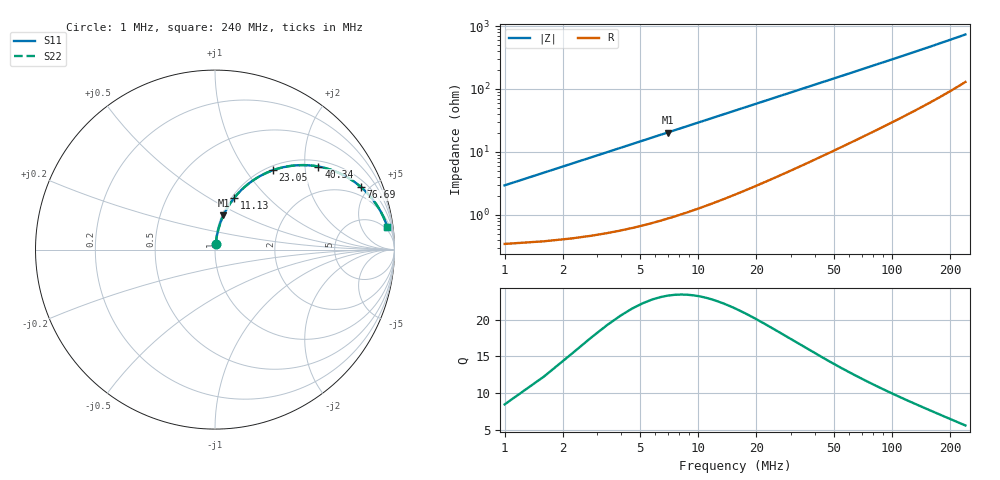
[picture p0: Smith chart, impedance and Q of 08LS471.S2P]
! Coilcraft 0805LS-471 Chip Inductor
! 18 September 2002
# MHZ S MA R 50
!Freq  MagS11  AngS11  MagS21  AngS21  MagS12  AngS12  MagS22  AngS22
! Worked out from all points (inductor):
!   403 points, 1 MHz to 240 MHz, reference 50 ohm
!   read as one part in series: L = 465 nH near 2.192 MHz
!   highest Q = 23.3 at 6.96 MHz (marker M1), where L = 465 nH
!   S11 on the Smith chart (normalised r, x): 1 MHz: 1.01, +0.06; 11.13 MHz: 1.03, +0.65; 23.05 MHz: 1.07, +1.34; 40.34 MHz: 1.15, +2.35; 76.69 MHz: 1.39, +4.48; 240 MHz: 4, +14
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1  0.0293 81.6  0.9961 -1.7  0.9961 -1.7  0.0293 81.6
1.596  0.04654 82.7  0.9951 -2.7  0.9951 -2.7  0.04654 82.7
2.788  0.08091 82.1  0.9921 -4.6  0.9921 -4.6  0.08091 82.1
3.98  0.1149 80.6  0.9878 -6.6  0.9878 -6.6  0.1149 80.6
5.172  0.1485 78.9  0.9823 -8.5  0.9823 -8.5  0.1485 78.9
6.96  0.1977 76.2  0.9718 -11.4  0.9718 -11.4  0.1977 76.2
8.748  0.2451 73.4  0.9591 -14.2  0.9591 -14.2  0.2451 73.4
11.132  0.3054 69.7  0.939 -17.8  0.939 -17.8  0.3054 69.7
16.496  0.4263 62.1  0.8847 -25.2  0.8847 -25.2  0.4263 62.1
23.052  0.5455 54.0  0.8102 -33.0  0.8102 -33.0  0.5455 54.0
30.8  0.6503 46.2  0.7229 -40.5  0.7229 -40.5  0.6503 46.2
40.336  0.7393 38.8  0.6273 -47.5  0.6273 -47.5  0.7393 38.8
40.932  0.7437 38.4  0.6218 -47.9  0.6218 -47.9  0.7437 38.4
48.68  0.7924 33.7  0.5568 -52.2  0.5568 -52.2  0.7924 33.7
57.024  0.8304 29.8  0.4979 -55.9  0.4979 -55.9  0.8304 29.8
76.692  0.8855 23.1  0.394 -61.9  0.394 -61.9  0.8855 23.1
80.864  0.8933 22.0  0.3767 -62.8  0.3767 -62.8  0.8933 22.0
98.744  0.9179 18.3  0.3162 -66.0  0.3162 -66.0  0.9179 18.3
120.796  0.9363 15.1  0.2626 -68.5  0.2626 -68.5  0.9363 15.1
160.728  0.9542 11.4  0.1992 -71.1  0.1992 -71.1  0.9542 11.4
200.66  0.9632 9.0  0.1591 -72.2  0.1591 -72.2  0.9632 9.0
240  0.9683 7.5  0.1319 -72.4  0.1319 -72.4  0.9683 7.5
